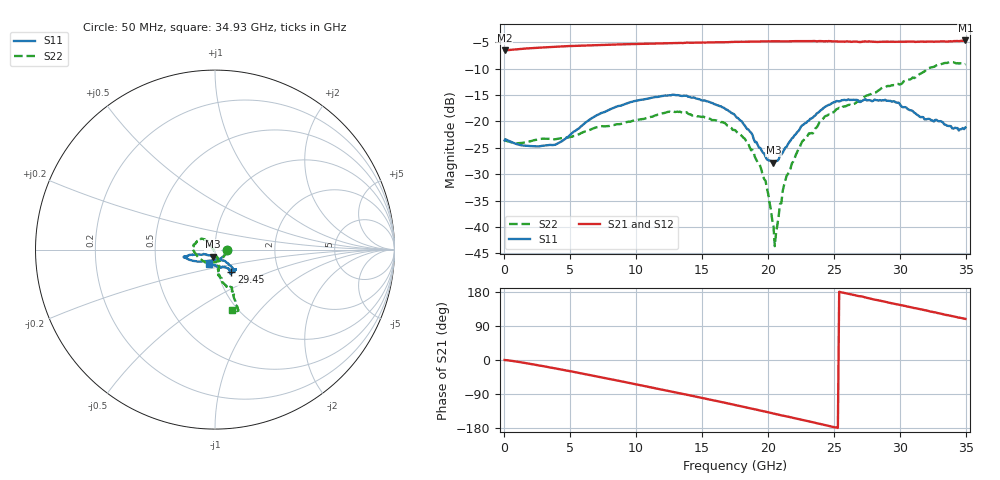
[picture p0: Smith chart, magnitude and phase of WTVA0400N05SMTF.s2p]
! 50 ohm 2-Port S-parameters measured by Modelithics Inc support@modelithics.com  Tampa, FL USA 813-866-6335 (February 2024)
! Smiths Interconnect,  4dB P/N: WTVA0400N05SMTF, Temperature: -50 C
! Board: 10 mil Rogers 4350B, Mounting Pad Dimensions: Length: 15 mils, Width: 25 mils, Gap: 40 mils.
# Hz S RI R 50
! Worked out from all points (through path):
!   352 points, 50 MHz to 34.93 GHz, reference 50 ohm
!   highest |S21| = -4.65 dB at 34.93 GHz (marker M1); lowest = -6.5 dB at 50 MHz (marker M2)
!   group delay of S21, straight-line fit = 20.5 ps
!   lowest |S11| = -27.8 dB at 20.4 GHz (marker M3), VSWR 1.08, Z = 48.7 - j3.78 ohm
!   |S11| at or under -10 dB: start of sweep to end of sweep
!   |S22| runs from -43.6 to -8.8 dB; largest |S21 - S12| = 0.0035
!   S11 on the Smith chart (normalised r, x): 50 MHz: 1.14, -0.01; 29.45 GHz: 1.16, -0.30; 34.93 GHz: 0.92, -0.15
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5e7  0.066 -0.00233  0.4716 -0.000379  0.4715 -0.000662  0.0673 -0.00227
3.8815e9  -0.00829 -0.0595  0.4728 -0.1919  0.4724 -0.1921  0.0106 -0.067
5.8715e9  -0.0632 -0.0649  0.427 -0.3038  0.4268 -0.3039  -0.0282 -0.0726
8.4585e9  -0.1221 -0.0629  0.3204 -0.4301  0.3199 -0.43  -0.0712 -0.0607
1.1742e10  -0.1664 -0.0441  0.1276 -0.5333  0.1269 -0.5333  -0.1161 -0.0121
1.38315e10  -0.1709 -0.04  -0.0144 -0.5583  -0.0145 -0.5581  -0.1192 0.0275
1.7513e10  -0.1102 -0.0264  -0.2749 -0.4979  -0.2751 -0.4976  -0.0594 0.0572
1.84085e10  -0.0797 -0.0283  -0.3325 -0.4625  -0.3322 -0.4626  -0.0437 0.0475
1.94035e10  -0.0475 -0.0298  -0.392 -0.4153  -0.3924 -0.4147  -0.0265 0.0264
1.98015e10  -0.0339 -0.0313  -0.4167 -0.3949  -0.4162 -0.3952  -0.0205 0.018
2.03985e10  -0.0119 -0.0387  -0.4483 -0.3608  -0.4484 -0.3604  -0.0103 0.00016
2.0498e10  -0.00819 -0.0405  -0.4535 -0.3549  -0.4537 -0.3543  -0.00592 -0.00285
2.0896e10  0.00875 -0.0468  -0.4718 -0.3276  -0.4717 -0.3274  -0.00189 -0.0164
2.09955e10  0.0109 -0.0473  -0.4746 -0.3215  -0.4747 -0.3211  0.000407 -0.0168
2.13935e10  0.0215 -0.0533  -0.4907 -0.2983  -0.4909 -0.2978  0.00461 -0.0301
2.25875e10  0.0614 -0.0686  -0.5349 -0.2151  -0.5349 -0.2147  0.0181 -0.0625
2.33835e10  0.0746 -0.0795  -0.5558 -0.1569  -0.5557 -0.1567  0.0169 -0.0753
2.51745e10  0.108 -0.113  -0.5743 -0.0157  -0.5742 -0.0157  0.0231 -0.1287
2.91545e10  0.0851 -0.1312  -0.4982 0.2744  -0.4978 0.2748  0.0655 -0.2061
2.9453e10  0.0911 -0.1256  -0.4887 0.2933  -0.4879 0.2944  0.0756 -0.2076
3.2836e10  0.0231 -0.0984  -0.3183 0.4753  -0.3195 0.4743  0.1246 -0.3223
3.49255e10  -0.0338 -0.0808  -0.1853 0.5556  -0.183 0.5562  0.0956 -0.336
